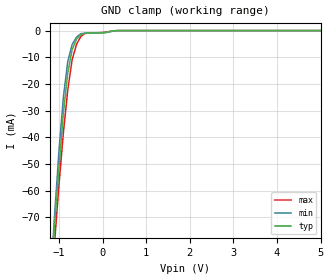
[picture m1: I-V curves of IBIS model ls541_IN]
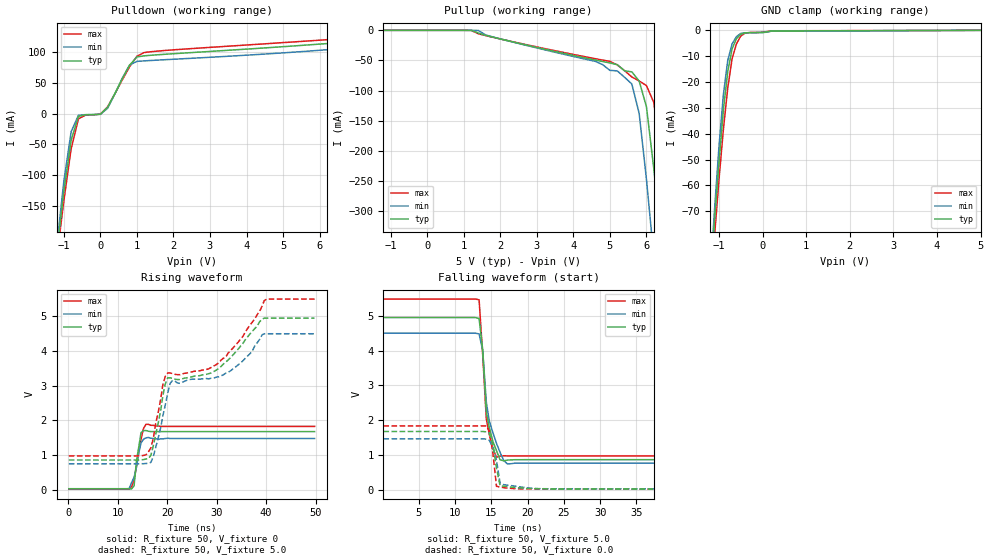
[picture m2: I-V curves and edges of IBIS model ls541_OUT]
| TEXAS INSTRUMENTS INCORPORATED
| Standard Linear and Logic Group
| IBIS Model of SN74LS541
| OCTAL BUFFERS AND LINE DRIVERS WITH 3-STATE OUTPUTS
| SOIC 20-pin (DW),SOP 20-pin (NS), SSOP 20-pin (DB), Packages.
[IBIS Ver]   3.2
[Comment Char]  |_char
[File Name]   sn74ls541.ibs
[File Rev]   2.1 I_die
[Date]   Nov. 22, 2004
[Source]   File originated at Texas Instruments, Inc.
[Notes]   The following is a sample IBIS file for the LS541.
   - FILE REV HISTORY
   - 2.1 Re-Release IBIS file on 11/22/04
   - Power clamp data deleted as there is no power-clamp diode.
|   - All test data contained in this file are derived from
|   actual measurements.
|   - File created by Nobuhisa Ohtsubo, SLL Product Engineering.
[Disclaimer] Property of Texas Instruments Incorporated.  Unauthorized
   reproduction and/or distribution is strictly prohibited.
   This product is protected under copyright law.
   Created 2000, (C) Copyright 2000, Texas Instruments Inc.,
   All Rights Reserved.
   UNLESS THERE IS A SIGNED, WRITTEN AGREEMENT TO THE
   CONTRARY, TEXAS INSTRUMENTS () IS PROVIDING THE IBIS
   MODELS  AND WITHOUT ANY WARRANTY, EXPRESSED OR
   IMPLIED.  TI assumes no liability for:
   1) the accuracy of the IBIS models provided to your
   company;
   2) the proper functioning of these IBIS Models in your
   design or for any resulting applications; or
   3) infringement of patents, copyrights or intellectual
   property rights resulting from your use of these IBIS
   models.
   TI provides IBIS Models as a service to our customers.
   You and your company shall not distribute, sell or give
   these models to anyone else without prior written
   permission from TI.
   TI reserves the right to make changes to our products or
   to discontinue any semiconductor product or service
   without notice, and advises our customers to obtain the
   latest version of relevant information to verify, before
   placing orders, that the information being relied on is
   current.
   Please be aware that your receipt and use of the IBIS
   information provided shall serve as acceptance of these
   terms and conditions.  If you do not accept these terms,
   you should return or destroy the IBIS models and any
   other accompanying information immediately.
|   Component LS541_DW
[Component]   ls541_DW
[Manufacturer]  Texas Instruments, Inc.
[Package]
|   typ   min   max
R_pkg   0.038   0.033   0.045
L_pkg   5.012nH   4.110nH   6.349nH
C_pkg   0.717pF   0.530pF   0.868pF
[Pin]   signal_name   model_name   R_pin   L_pin   C_pin
1   G1_NOT   ls541_IN   0.042   6.336nH   0.865pF
2   A1   ls541_IN   0.043   5.542nH   0.867pF
3   A2   ls541_IN   0.034   4.714nH   0.732pF
4   A3   ls541_IN   0.034   4.377nH   0.591pF
5   A4   ls541_IN   0.036   4.130nH   0.533pF
6   A5   ls541_IN   0.035   4.111nH   0.530pF
7   A6   ls541_IN   0.034   4.284nH   0.583pF
8   A7   ls541_IN   0.034   4.634nH   0.726pF
9   A8   ls541_IN   0.040   5.518nH   0.865pF
10   GND   GND   0.043   6.349nH   0.866pF
11   Y8   ls541_OUT   0.041   6.281nH   0.861pF
12   Y7   ls541_OUT   0.045   5.561nH   0.868pF
13   Y6   ls541_OUT   0.033   4.778nH   0.742pF
14   Y5   ls541_OUT   0.035   4.414nH   0.596pF
15   Y4   ls541_OUT   0.035   4.110nH   0.533pF
16   Y3   ls541_OUT   0.036   4.130nH   0.533pF
17   Y2   ls541_OUT   0.034   4.377nH   0.591pF
18   Y1   ls541_OUT   0.034   4.714nH   0.731pF
19   G2_NOT   ls541_IN   0.043   5.569nH   0.868pF
20   VCC   POWER   0.042   6.308nH   0.864p
|   Component LS541_NS
[Component]   ls541_NS
[Manufacturer]  Texas Instruments, Inc.
[Package]
|   typ   min   max
R_pkg   0.044   0.029   0.058
L_pkg   3.666nH   2.317nH   5.115nH
C_pkg   0.548pF   0.316pF   0.725pF
[Pin]   signal_name   model_name   R_pin   L_pin   C_pin
1   G1_NOT   ls541_IN   0.058   5.115nH   0.725pF
2   A1   ls541_IN   0.053   4.591nH   0.724pF
3   A2   ls541_IN   0.049   3.754nH   0.572pF
4   A3   ls541_IN   0.029   2.549nH   0.388pF
5   A4   ls541_IN   0.031   2.317nH   0.316pF
6   A5   ls541_IN   0.031   2.317nH   0.316pF
7   A6   ls541_IN   0.029   2.556nH   0.399pF
8   A7   ls541_IN   0.049   3.754nH   0.579pF
9   A8   ls541_IN   0.053   4.591nH   0.724pF
10   GND   GND   0.058   5.115nH   0.725pF
11   Y8   ls541_OUT   0.058   5.115nH   0.725pF
12   Y7   ls541_OUT   0.053   4.591nH   0.724pF
13   Y6   ls541_OUT   0.049   3.754nH   0.579pF
14   Y5   ls541_OUT   0.029   2.557nH   0.399pF
15   Y4   ls541_OUT   0.031   2.317nH   0.316pF
16   Y3   ls541_OUT   0.031   2.317nH   0.316pF
17   Y2   ls541_OUT   0.029   2.557nH   0.399pF
18   Y1   ls541_OUT   0.049   3.754nH   0.579pF
19   G2_NOT   ls541_IN   0.053   4.591nH   0.724pF
20   VCC   POWER   0.058   5.115nH   0.725pF
|   Component LS541_DB
[Component]   ls541_DB
[Manufacturer]  Texas Instruments, Inc.
[Package]
|   typ   min   max
R_pkg   0.040   0.035   0.051
L_pkg   3.495nH   3.035nH   4.314nH
C_pkg   0.420pF   0.346pF   0.502pF
[Pin]   signal_name   model_name   R_pin   L_pin   C_pin
1   G1_NOT   ls541_IN   0.049   4.310nH   0.502pF
2   A1   ls541_IN   0.048   3.903nH   0.487pF
3   A2   ls541_IN   0.035   3.189nH   0.396pF
4   A3   ls541_IN   0.035   3.036nH   0.347pF
5   A4   ls541_IN   0.035   3.035nH   0.367pF
6   A5   ls541_IN   0.035   3.035nH   0.367pF
7   A6   ls541_IN   0.035   3.036nH   0.347pF
8   A7   ls541_IN   0.035   3.189nH   0.397pF
9   A8   ls541_IN   0.047   3.899nH   0.488pF
10   GND   GND   0.051   4.314nH   0.500pF
11   Y1   ls541_OUT   0.051   4.314nH   0.500pF
12   Y2   ls541_OUT   0.047   3.899nH   0.488pF
13   Y3   ls541_OUT   0.035   3.189nH   0.397pF
14   Y4   ls541_OUT   0.035   3.036nH   0.346pF
15   Y5   ls541_OUT   0.035   3.035nH   0.367pF
16   Y6   ls541_OUT   0.035   3.035nH   0.367pF
17   Y7   ls541_OUT   0.035   3.036nH   0.346pF
18   Y8   ls541_OUT   0.035   3.189nH   0.397pF
19   G2_NOT   ls541_IN   0.047   3.899nH   0.488pF
20   VCC   POWER   0.051   4.314nH   0.502pF
| Models and submodels in the file (2): ls541_IN (Input), ls541_OUT (3-state)
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|   Model LS541_IN
[Model]   ls541_IN
Model_type  Input
Polarity   Inverting
Vinl = 0.8
Vinh = 2.0
| variable   typ   min   max
C_comp   1.33pf   1.00pf   1.66pf
[Temperature Range]   25   0   70
[Voltage Range]   5.0   4.75   5.25
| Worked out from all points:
|   GND clamp passes 1 mA (typ) near -0.41 V on its own axis
[GND Clamp]
|   Voltage   I(typ)   I(min)   I(max)
-5V       -1.19A     -1.28A     -1.1A
-1.2V     -97.9mA    -94.9mA    -103mA
-1.1V     -73mA      -68.8mA    -79.1mA
-1V       -51.2mA    -44.9mA    -57.6mA
-900mV    -30.9mA    -25mA      -38.4mA
-800mV    -16mA      -11.7mA    -22.4mA
-700mV    -7.17mA    -5.25mA    -11mA
-600mV    -3.23mA    -2.46mA    -5.25mA
-500mV    -1.49mA    -1.17mA    -2.19mA
-400mV    -972uA     -958uA     -1.08mA
300mV     -31.8uA    -42.7uA    -27.7uA
5V        848pA      59.6pA     3.3nA
|   Model LS541_OUT
[Model]   ls541_OUT
Model_type  3-state
Polarity   Non-Inverting
Enable   Active-Low
Vmeas = 1.3v
Cref = 0pf
| variable   typ   min   max
C_comp   5.8pf   4.35pf   7.25pf
[Temperature Range]   25   0   70
[Voltage Range]   5.0   4.5   5.5
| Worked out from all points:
|   slope of the pulldown table from 0 to 0.75 V, typ, clamps not added: 10.2 ohm
|   GND clamp passes 1 mA (typ) near -0.41 V on its own axis
|   rising waveform, R_fixture 50, V_fixture 0: 20-80 % time 914ps typ, 1.28ns min, 1.29ns max; typ from 0.031 V to 1.68 V
|   falling waveform, R_fixture 50, V_fixture 5.0: 20-80 % time 1.1ns typ, 1.53ns min, 869ps max; typ from 4.95 V to 0.871 V
|   rising waveform, R_fixture 50, V_fixture 5.0: 20-80 % time 17ns typ, 17.3ns min, 18.4ns max; typ from 0.86 V to 4.95 V
|   falling waveform, R_fixture 50, V_fixture 0.0: 20-80 % time 826ps typ, 839ps min, 678ps max; typ from 1.68 V to 0.032 V
[Pulldown]
|   Voltage   I(typ)   I(min)   I(max)
-5V       -2.251A    -2.394A    -2.101A
-1.2V     -228.3mA   -218.6mA   -236.3mA
-1V       -125.8mA   -109.7mA   -141.3mA
-800mV    -43.31mA   -29.43mA   -57.06mA
-600mV    -4.546mA   -2.797mA   -8.615mA
0V        -1.168mA   -1.308mA   -1.051mA
200mV     10.18mA    8.496mA    11.05mA
800mV     78.07mA    78.39mA    75.4mA
1V        91.36mA    84.23mA    92.47mA
1.4V      94.2mA     85.75mA    99.96mA
5.6V      110.5mA    100.4mA    116.9mA
10V       131.3mA    124.3mA    139.6mA
[Pullup]
|   Voltage   II(typ)   I(min)   I(max)
-5V       2.11uA     674.1nA    5.805uA
1.4V      -4.41mA    -283.6uA   -5.664mA
4.6V      -49.31mA   -51.51mA   -47.11mA
5V        -54.19mA   -66.44mA   -51.67mA
5.2V      -56.96mA   -67.32mA   -57.4mA
5.6V      -68.94mA   -89.12mA   -77.47mA
5.8V      -84.15mA   -137.7mA   -84.06mA
6V        -126.8mA   -247.3mA   -91.78mA
6.2V      -228.9mA   -374.8mA   -119.5mA
6.4V      -345.4mA   -478.1mA   -213.4mA
6.6V      -442.7mA   -589.6mA   -319.5mA
10V       -2.246A    -2.52A     -1.968A
[GND Clamp]
|   Voltage   I(typ)   I(min)   I(max)
-5V       -1.19A     -1.28A     -1.1A
-1.2V     -97.9mA    -94.9mA    -103mA
-1.1V     -73mA      -68.8mA    -79.1mA
-1V       -51.2mA    -44.9mA    -57.6mA
-900mV    -30.9mA    -25mA      -38.4mA
-800mV    -16mA      -11.7mA    -22.4mA
-700mV    -7.17mA    -5.25mA    -11mA
-600mV    -3.23mA    -2.46mA    -5.25mA
-500mV    -1.49mA    -1.17mA    -2.19mA
-400mV    -972uA     -958uA     -1.08mA
200mV     -247uA     -329uA     -190uA
5V        848pA      59.6pA     3.3nA
[Ramp]
| variable   typ   min   max
dV/dt_r   1.284/1.314n   1.056/1.149n   1.518/1.587n
dV/dt_f   2.742/1.529n   2.448/2.041n   3.042/1.254n
R_load = 50
[Rising Waveform]
R_fixture = 50
V_fixture = 0
|   Time   V(typ)   V(min)   V(max)
97.7ps    30.8mV     33.2mV     21.2mV
12.3ns    30mV       38.1mV     20.3mV
12.8ns    30mV       213mV      94.6mV
13.3ns    121mV      362mV      280mV
13.8ns    860mV      668mV      700mV
14.7ns    1.65V      1.35V      1.46V
15.2ns    1.71V      1.46V      1.77V
15.7ns    1.71V      1.5V       1.89V
18.7ns    1.68V      1.47V      1.83V
49.8ns    1.68V      1.48V      1.83V
[Falling Waveform]
R_fixture = 50
V_fixture = 5.0
V_fixture_min = 4.5
V_fixture_max = 5.5
|   Time   V(typ)   V(min)   V(max)
97.7ps    4.95V      4.5V       5.48V
13.3ns    4.92V      4.48V      5.46V
13.8ns    4.02V      4V         3.87V
14.3ns    2.24V      2.52V      2.04V
14.7ns    1.8V       1.99V      1.6V
15.2ns    1.4V       1.65V      1.19V
15.7ns    1.13V      1.34V      942mV
16.2ns    866mV      1.08V      974mV
17.2ns    860mV      752mV      980mV
49.8ns    871mV      770mV      980mV
[Rising Waveform]
R_fixture = 50
V_fixture = 5.0
V_fixture_min = 4.5
V_fixture_max = 5.5
|   Time   V(typ)   V(min)   V(max)
97.7ps    860mV      752mV      980mV
15.7ns    889mV      760mV      1.01V
17.2ns    1.28V      970mV      1.5V
19.1ns    2.7V       2.12V      3.02V
20.1ns    3.23V      2.79V      3.37V
21.1ns    3.21V      3.16V      3.35V
30.4ns    3.5V       3.26V      3.66V
34.8ns    4.14V      3.65V      4.34V
40.1ns    4.95V      4.5V       5.5V
49.8ns    4.95V      4.5V       5.5V
[Falling Waveform]
R_fixture = 50
V_fixture = 0.0
|   Time   V(typ)   V(min)   V(max)
97.7ps    1.68V      1.47V      1.84V
14.3ns    1.67V      1.46V      1.84V
14.7ns    1.64V      1.43V      1.7V
15.2ns    1.31V      1.23V      1.07V
15.7ns    633mV      860mV      108mV
16.2ns    120mV      191mV      82.4mV
16.7ns    110mV      154mV      67.9mV
19.1ns    60.2mV     85mV       32.9mV
21.6ns    36mV       39mV       27.2mV
49.8ns    32mV       35mV       24.9mV
